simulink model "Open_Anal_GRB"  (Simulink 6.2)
settings: Solver=ode5  StartTime=0.0  StopTime=25000  FixedStep=Tsr  RelTol=1e-3
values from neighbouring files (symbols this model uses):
  d2r = pi/180    (= 0.0174532925199)    [start.m]    (also in run.m; runf.m; orbitic.m; Quan.m)
  Kq1 = I22*ww^2 - 3*wo2*(I11-I33)    [start.m]    (also in run.m)
  Kq2 = 2*I22*zet*ww    [start.m]    (also in run.m)
  Kqi = 0.0005    [start.m]    (also in run.m)
  Kr1 = (0.1*I11*I33*zet^2/Hy0) - sqrt( ((0.01^zet^4*I11^2*I33^2)/Hy0^2)+(4*I11*I33*zet^2) )    [start.m]    (also in run.m)
  Kr2 = 0.05*Kr1    [start.m]    (also in run.m)
  Kr3 = 0.04*zet*(Kr2-Hy0) * sqrt(abs(Hy0/(I11*I33)))    [start.m]    (also in run.m)
  Ts = 0.01    [start.m]    (also in run.m = 0.001; runf.m = 0.0005)
  Tsr = 0.01    [start.m]
  wo = 0.00113    [start.m]    (also in run.m)
undefined symbols (not defined in the file or in its folder): Agr, Bgr, Cgr, den, Dgr, DiscIntNeverNeededParam, dsen, nsen, num, RW_Steering
libraries: simulink x4

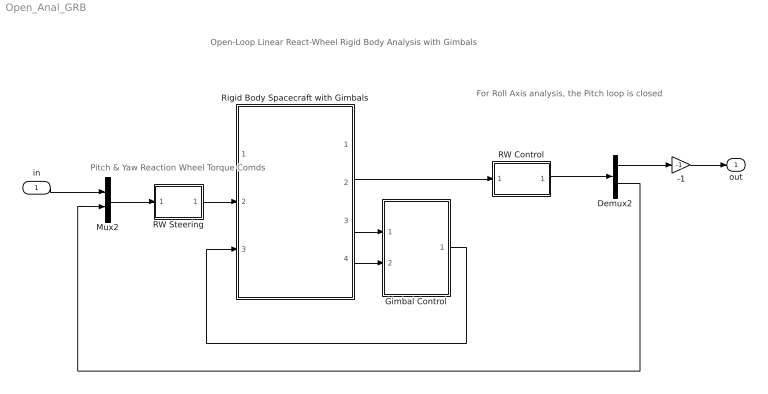
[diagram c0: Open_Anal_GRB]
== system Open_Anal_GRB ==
  note: Open-Loop Linear React-Wheel Rigid Body Analysis with Gimbals
  note: For Roll Axis analysis, the Pitch loop is closed
  note: Pitch & Yaw Reaction Wheel Torque Comds
  in : Inport  Port=1  LatchInput=off
  -1 : Gain  Gain=-1
  Demux2 : Demux  Outputs=2
  Gimbal Control : Subsystem
  Mux2 : Mux  Inputs=2
  RW Control : Subsystem
  RW Steering : Subsystem
  Rigid Body Spacecraft with Gimbals : Subsystem
  out : Outport
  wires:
  -1/1 -> out/1
  Mux2/1 -> RW Steering/1(Trwc)
  RW Control/1(Tc) -> Demux2/1
  Gimbal Control/1(GTrq) -> Rigid Body Spacecraft with Gimbals/3(Tgimb)
  Rigid Body Spacecraft with Gimbals/3(alfa) -> Gimbal Control/1(Gimb)
  Rigid Body Spacecraft with Gimbals/4(alfad) -> Gimbal Control/2(Grate)
  RW Steering/1(Twi) -> Rigid Body Spacecraft with Gimbals/2(Trw(i))
  Rigid Body Spacecraft with Gimbals/2(atti) -> RW Control/1(atti)
  Demux2/2 -> Mux2/2
  Demux2/1 -> -1/1
  in/1 -> Mux2/1

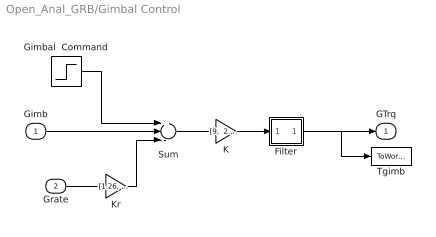
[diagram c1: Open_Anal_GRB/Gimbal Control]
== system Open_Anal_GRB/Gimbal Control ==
  Gimb : Inport  Port=1  LatchInput=off
  Grate : Inport  Port=2  LatchInput=off
  Filter : Subsystem
  Gimbal  Command : Step  After=[5, 5]*d2r  SampleTime=0
  K : Gain  Gain="[9,  2.85]"
  Kr : Gain  Gain="[1.26,  1.14]"
  Sum : Sum  Inputs=+--
  Tgimb : ToWorkspace  VariableName=Tgimb  SampleTime=-1  SaveFormat=Array
  GTrq : Outport
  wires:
  Sum/1 -> K/1
  Gimb/1 -> Sum/2
  Grate/1 -> Kr/1
  K/1 -> Filter/1(I)
  Kr/1 -> Sum/3
  Gimbal  Command/1 -> Sum/1
  Filter/1(O) -> GTrq/1, Tgimb/1

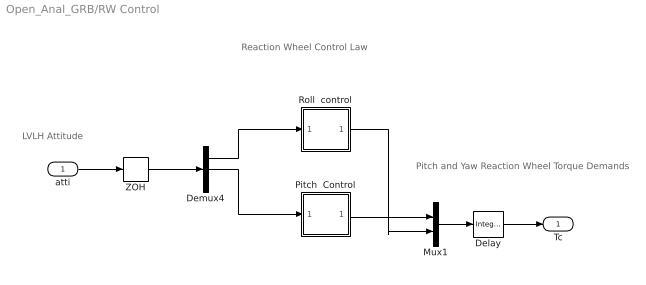
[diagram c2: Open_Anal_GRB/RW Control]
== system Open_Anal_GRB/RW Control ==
  note: Pitch and Yaw Reaction Wheel Torque Demands
  note: LVLH Attitude
  note: Reaction Wheel Control Law
  atti : Inport  Port=1  LatchInput=off
  Delay : simulink/Discrete/Integer Delay  vinit=0.0  samptime=Tsr  NumDelays=1
  Demux4 : Demux  Outputs=3
  Mux1 : Mux  Inputs=2
  Pitch  Control : Subsystem
  Roll  control : Subsystem
  ZOH : ZeroOrderHold  SampleTime=Tsr
  Tc : Outport
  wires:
  ZOH/1 -> Demux4/1
  Demux4/1 -> Roll  control/1(phi)
  Pitch  Control/1(Tcy) -> Mux1/1
  Demux4/2 -> Pitch  Control/1(the)
  atti/1 -> ZOH/1
  Mux1/1 -> Delay/1
  Roll  control/1(Tcz) -> Mux1/2
  Delay/1 -> Tc/1

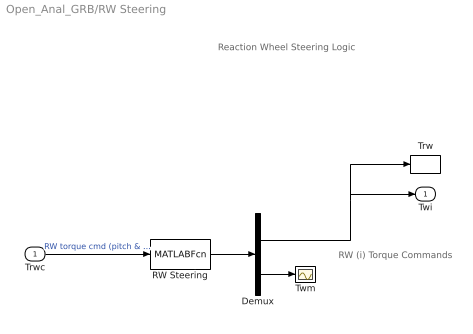
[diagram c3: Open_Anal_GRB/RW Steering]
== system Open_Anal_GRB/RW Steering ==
  note: RW (i) Torque Commands
  note: Reaction Wheel Steering Logic
  Trwc : Inport  Port=1  LatchInput=off
  Demux : Demux  Outputs=[2, 1]
  RW Steering : MATLABFcn  MATLABFcn=RW_Steering( u(1:2) )  OutputDimensions=3
  Trw : ToWorkspace  VariableName=Trw  SampleTime=-1  SaveFormat=Array
  Twm : Scope
  Twi : Outport
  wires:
  Demux/2 -> Twm/1
  Demux/1 -> Twi/1, Trw/1
  RW Steering/1 -> Demux/1
  Trwc/1 -> RW Steering/1  "RW torque cmd (pitch & yaw)"

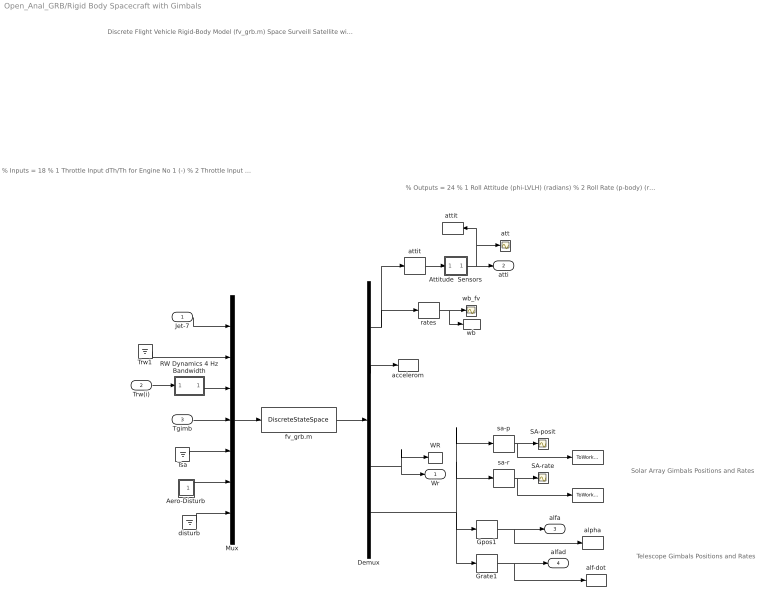
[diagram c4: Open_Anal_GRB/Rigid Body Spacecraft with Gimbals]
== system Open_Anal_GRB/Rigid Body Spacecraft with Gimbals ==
  note: % Inputs = 18 % 1 Throttle Input dTh/Th for Engine No 1 (-) % 2 Throttle Input dTh/Th for Engine No 2 (-) % 3 Throttle Input dTh/Th for Engine No 3 (-) % 4 Throttle Input dTh/Th for Engine No 4 (-) % 5 Throttle Input dTh/Th for Engine No 5 (-) % 6 Throttle Input dTh/Th for Engine No 6 (-) % 7 Throttle Input dTh/Th for Engine No 7 (-) % 8 Reaction Wheel No 1 Input Torque (ft-lb) % 9 Reaction Wheel No 2 Input Torque (ft-lb) % 10 Reaction Wheel No 3 Input Torque (ft-lb) % 11 Gimbaling Appendage Hinge # 1 Torque (ft-lb) % 12 Gimbaling Appendage Hinge # 2 Torque (ft-lb) % 13 Gimbaling Appendage Hinge # 3 Torque (ft-lb) % 14 Gimbaling Appendage Hinge # 4 Torque (ft-lb) % 15 External Torque Input 1 (ft-lb), direct: % 16 External Torque Input 2 (ft-lb), direct: % 17 External Torque Input 3 (ft-lb), direct: % 18 Ext Torque Direct.=( 0.1970 -0.5964 -0.7782)
  note: % Outputs = 24 % 1 Roll Attitude (phi-LVLH) (radians) % 2 Roll Rate (p-body) (rad/sec) % 3 Pitch Attitude (thet-LVLH) (radians) % 4 Pitch Rate (q-body) (rad/sec) % 5 Yaw Attitude (psi-LVLH) (radians) % 6 Yaw Rate (r-body) (rad/sec) % 7 Angle of attack, alfa, (radians) % 8 Angle of sideslip, beta, (radian) % 9 Change in Altitude, delta-h, (feet) % 10 Forward Acceleration (V-dot) (ft/sec) % 11 Cross Range Velocity (Vcr) (ft/sec) % 12 Accelerom # 1, (along X), (ft/sec^2) Translat. Acceler % 13 Accelerom # 2, (along Y), (ft/sec^2) Translat. Acceler % 14 Reaction Wheel # 1 Rate (rpm) relative to vehicle % 15 Reaction Wheel # 2 Rate (rpm) relative to vehicle % 16 Reaction Wheel # 3 Rate (rpm) relative to vehicle % 17 Gimbaling Appendage # 1 Relative Rotation, alfar( 1), % 18 Gimbaling Appendage # 1 Relative Rot.Rate, alfar-dot( % 19 Gimbaling Appendage # 2 Relative Rotation, alfar( 2), % 20 Gimbaling Appendage # 2 Relative Rot.Rate, alfar-dot( % 21 Gimbaling Appendage # 3 Relative Rotation, alfar( 3), % 22 Gimbaling Appendage # 3 Relative Rot.Rate, alfar-dot( % 23 Gimbaling Appendage # 4 Relative Rotation, alfar( 4), % 24 Gimbaling Appendage # 4 Relative Rot.Rate, alfar-dot(
  note: Discrete Flight Vehicle Rigid-Body Model (fv_grb.m) Space Surveill Satellite with RCS and Reaction Wheels (Gimbals, No Flex, Z-Transf)
  note: Telescope Gimbals Positions and Rates
  note: Solar Array Gimbals Positions and Rates
  Jet-7 : Inport  Port=1  LatchInput=off
  Trw(i) : Inport  Port=2  LatchInput=off
  Tgimb : Inport  Port=3  LatchInput=off
  " " : ToWorkspace  VariableName=SA_pos  SampleTime=-1  SaveFormat=Array
  "   " : ToWorkspace  VariableName=SA_rate  SampleTime=-1  SaveFormat=Array
  Aero-Disturb : Subsystem
  Attitude  Sensors : Subsystem
  Demux : Demux  Outputs=[11, 2, 1,2, 8]
  Gpos1 : Selector  Elements=[1,3]  InputPortWidth=8
  Grate1 : Selector  Elements=[2, 4]  InputPortWidth=8
  Mux : Mux  Inputs=[7, 1,2, 2,2, 3,1]
  RW Dynamics 4 Hz Bandwidth : Subsystem
  SA-posit : Scope
  SA-rate : Scope
  Trw1 : Ground
  Tsa : Ground
  WR : ToWorkspace  VariableName=wr  SampleTime=-1  SaveFormat=Array
  accelerom : ToWorkspace  VariableName=accel  SampleTime=-1  SaveFormat=Array
  alf-dot : ToWorkspace  VariableName=alfad  SampleTime=-1  SaveFormat=Array
  alpha : ToWorkspace  VariableName=alfa  SampleTime=-1  SaveFormat=Array
  att : Scope
  attit : Selector  Elements=[1, 3, 5]  InputPortWidth=11
  "attit " : ToWorkspace  VariableName=atti  SampleTime=-1  SaveFormat=Array
  disturb : Ground
  fv_grb.m : DiscreteStateSpace  A=Agr  B=Bgr  C=Cgr  D=Dgr  SampleTime=Tsr
  rates : Selector  Elements=[2, 4, 6]  InputPortWidth=11
  sa-p : Selector  Elements=[5, 7]  InputPortWidth=8
  sa-r : Selector  Elements=[6, 8]  InputPortWidth=8
  wb : ToWorkspace  VariableName=wb  SampleTime=-1  SaveFormat=Array
  wb_fv : Scope
  Wr : Outport
  atti : Outport  Port=2
  alfa : Outport  Port=3
  alfad : Outport  Port=4
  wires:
  Demux/4 -> Wr/1, WR/1
  Demux/1 -> rates/1, attit/1
  rates/1 -> wb_fv/1, wb/1
  attit/1 -> Attitude  Sensors/1(I)
  Demux/2 -> accelerom/1
  Jet-7/1 -> Mux/1
  Trw(i)/1 -> RW Dynamics 4 Hz Bandwidth/1(I)
  Tgimb/1 -> Mux/4
  Aero-Disturb/1(Td) -> Mux/6
  disturb/1 -> Mux/7
  Tsa/1 -> Mux/5
  fv_grb.m/1 -> Demux/1
  Mux/1 -> fv_grb.m/1
  Trw1/1 -> Mux/2
  Attitude  Sensors/1(O) -> atti/1, att/1, "attit "/1
  RW Dynamics 4 Hz Bandwidth/1(O) -> Mux/3
  Demux/5 -> Gpos1/1, Grate1/1, sa-p/1, sa-r/1
  Grate1/1 -> alfad/1, alf-dot/1
  Gpos1/1 -> alfa/1, alpha/1
  sa-p/1 -> SA-posit/1, " "/1
  sa-r/1 -> SA-rate/1, "   "/1

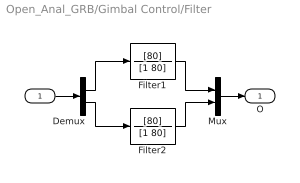
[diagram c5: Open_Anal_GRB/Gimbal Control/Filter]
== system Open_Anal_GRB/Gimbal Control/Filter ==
  I : Inport  Port=1  LatchInput=off
  Demux : Demux  Outputs=2
  Filter1 : TransferFcn  Numerator=[80]  Denominator=[1 80]
  Filter2 : TransferFcn  Numerator=[80]  Denominator=[1 80]
  Mux : Mux  Inputs=2
  O : Outport
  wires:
  Mux/1 -> O/1
  I/1 -> Demux/1
  Demux/2 -> Filter2/1
  Demux/1 -> Filter1/1
  Filter2/1 -> Mux/2
  Filter1/1 -> Mux/1

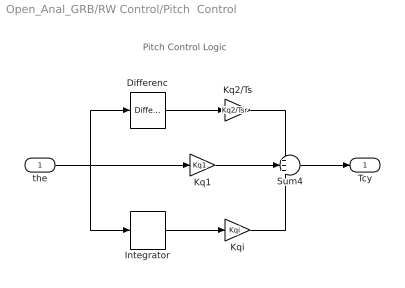
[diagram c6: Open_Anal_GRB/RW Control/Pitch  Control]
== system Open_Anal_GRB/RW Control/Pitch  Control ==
  note: Pitch Control Logic
  the : Inport  Port=1  LatchInput=off
  Differenc : simulink/Discrete/Difference  ICPrevInput=0.0  OutDataType=sfix(16)  OutScaling=2^-10  DoSatur=off
  Integrator : DiscreteIntegrator  SampleTime=Tsr  ICPrevOutput=DiscIntNeverNeededParam  ICPrevScaledInput=DiscIntNeverNeededParam
  Kq1 : Gain  Gain=Kq1
  Kq2/Ts : Gain  Gain=Kq2/Tsr
  Kqi : Gain  Gain=Kqi
  Sum4 : Sum  Inputs=+++
  Tcy : Outport
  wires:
  Kq1/1 -> Sum4/2
  Sum4/1 -> Tcy/1
  Kq2/Ts/1 -> Sum4/1
  the/1 -> Kq1/1, Integrator/1, Differenc/1
  Kqi/1 -> Sum4/3
  Integrator/1 -> Kqi/1
  Differenc/1 -> Kq2/Ts/1

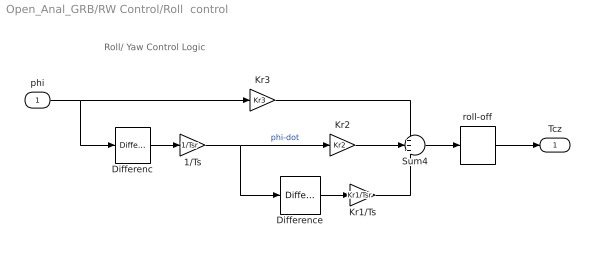
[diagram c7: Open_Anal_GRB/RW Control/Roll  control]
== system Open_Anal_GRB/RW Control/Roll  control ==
  note: Roll/ Yaw Control Logic
  phi : Inport  Port=1  LatchInput=off
  1/Ts : Gain  Gain=1/Tsr
  Differenc : simulink/Discrete/Difference  ICPrevInput=0.0  OutDataType=sfix(16)  OutScaling=2^-10  DoSatur=off
  Difference : simulink/Discrete/Difference  ICPrevInput=0.0  OutDataType=sfix(16)  OutScaling=2^-10  DoSatur=off
  Kr1/Ts : Gain  Gain=Kr1/Tsr
  Kr2 : Gain  Gain=Kr2
  Kr3 : Gain  Gain=Kr3
  Sum4 : Sum  Inputs=+++
  roll-off : DiscreteTransferFcn  Numerator=[num]  Denominator=[den]  SampleTime=Tsr
  Tcz : Outport
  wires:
  roll-off/1 -> Tcz/1
  Kr3/1 -> Sum4/1
  Kr2/1 -> Sum4/2
  Kr1/Ts/1 -> Sum4/3
  phi/1 -> Kr3/1, Differenc/1
  Sum4/1 -> roll-off/1
  Difference/1 -> Kr1/Ts/1
  Differenc/1 -> 1/Ts/1
  1/Ts/1 -> Kr2/1, Difference/1  "phi-dot"

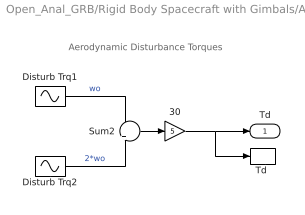
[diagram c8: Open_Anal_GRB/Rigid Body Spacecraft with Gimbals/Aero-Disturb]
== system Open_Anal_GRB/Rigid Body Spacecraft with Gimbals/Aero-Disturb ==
  note: Aerodynamic Disturbance Torques
  30 : Gain  Gain=5
  Disturb Trq1 : Sin  Amplitude="[0.0,   1,   0.2]*0.0001"  Bias="[0.0,  0.5,  0.15]*0.0001"  Frequency=[wo, wo, wo]  SampleTime=0
  Disturb Trq2 : Sin  Amplitude=[0, 1.2, 1]*0.0001  Bias=[0 0 0]  Frequency=[wo, wo, wo]*2  SampleTime=0
  Sum2 : Sum  Inputs=+|+
  "Td " : ToWorkspace  VariableName=Td  SampleTime=-1  SaveFormat=Array
  Td : Outport
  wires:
  30/1 -> "Td "/1, Td/1
  Disturb Trq2/1 -> Sum2/2  "2*wo"
  Sum2/1 -> 30/1
  Disturb Trq1/1 -> Sum2/1  "wo"

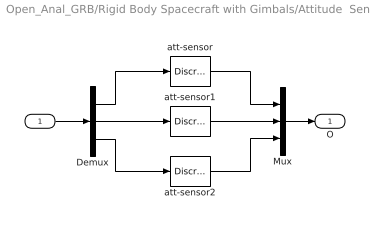
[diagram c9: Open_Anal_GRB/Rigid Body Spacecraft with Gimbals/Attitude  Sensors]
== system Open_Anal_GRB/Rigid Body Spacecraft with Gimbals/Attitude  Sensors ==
  I : Inport  Port=1  LatchInput=off
  Demux : Demux  Outputs=3
  Mux : Mux  Inputs=3
  att-sensor : DiscreteTransferFcn  Numerator=[nsen]  Denominator=[dsen]  SampleTime=Ts
  att-sensor1 : DiscreteTransferFcn  Numerator=[nsen]  Denominator=[dsen]  SampleTime=Ts
  att-sensor2 : DiscreteTransferFcn  Numerator=[nsen]  Denominator=[dsen]  SampleTime=Ts
  O : Outport
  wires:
  I/1 -> Demux/1
  Mux/1 -> O/1
  att-sensor/1 -> Mux/1
  Demux/1 -> att-sensor/1
  Demux/3 -> att-sensor2/1
  att-sensor2/1 -> Mux/3
  Demux/2 -> att-sensor1/1
  att-sensor1/1 -> Mux/2

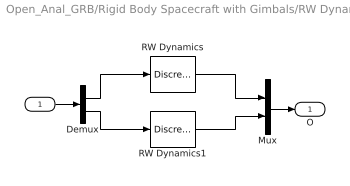
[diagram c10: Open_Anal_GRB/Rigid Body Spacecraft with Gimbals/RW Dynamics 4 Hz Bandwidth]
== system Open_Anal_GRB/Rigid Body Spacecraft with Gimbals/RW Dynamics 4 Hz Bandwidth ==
  I : Inport  Port=1  LatchInput=off
  Demux : Demux  Outputs=2
  Mux : Mux  Inputs=2
  RW Dynamics : DiscreteTransferFcn  Numerator="[0  0.221199217]"  Denominator=[1 -0.778800783]  SampleTime=Ts
  RW Dynamics1 : DiscreteTransferFcn  Numerator="[0  0.221199217]"  Denominator=[1 -0.778800783]  SampleTime=Ts
  O : Outport
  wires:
  Demux/2 -> RW Dynamics1/1
  Demux/1 -> RW Dynamics/1
  I/1 -> Demux/1
  Mux/1 -> O/1
  RW Dynamics/1 -> Mux/1
  RW Dynamics1/1 -> Mux/2
